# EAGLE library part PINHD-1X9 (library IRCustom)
Pin header 1x10 0.1" spacing With round pins
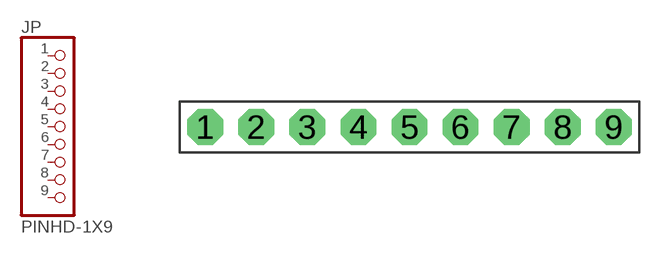
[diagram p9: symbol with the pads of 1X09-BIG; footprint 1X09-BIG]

Designator prefix JP

## PINHD-1X9  [1X09-BIG]
1  1  pas
2  2  pas
3  3  pas
4  4  pas
5  5  pas
6  6  pas
7  7  pas
8  8  pas
9  9  pas

## Footprint 1X09-BIG (pad centres in mm)
drill 1.016 pad 1.778 octagon: 1 -10.16,0; 2 -7.62,0; 3 -5.08,0; 4 -2.54,0; 5 0,0; 6 2.54,0; 7 5.08,0; 8 7.62,0; 9 10.16,0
